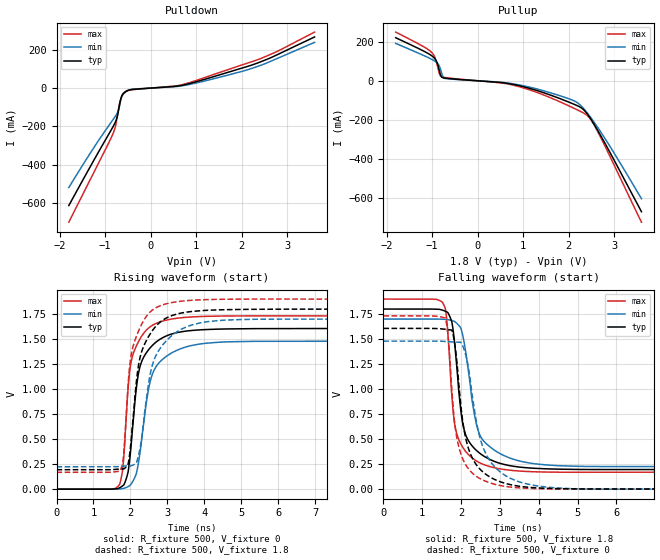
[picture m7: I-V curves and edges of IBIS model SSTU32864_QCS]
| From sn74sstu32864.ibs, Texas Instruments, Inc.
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[Model]   SSTU32864_QCS
Model_type  Output
Vref =   1.8
Rref =   1000
Cref =   30p
Vmeas =   0.9
| variable   typ   min   max
C_comp   4.54pF   3.63pF   5.50pF
| C_pullup   4.56pF   3.63pF   5.50pF
| C_pulldown   4.53pF   3.73pF   5.14pF
[Temperature Range]   40   85   0
| Ambient temperature   25   70   0
[Voltage range]   1.8   1.7   1.9
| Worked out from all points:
|   slope of the pulldown table from 0 to 0.27 V, typ, clamps not added: 60.6 ohm
|   slope of the pullup table from 0 to 0.27 V, typ, clamps not added: 59.5 ohm
|   rising waveform, R_fixture 500, V_fixture 0: 20-80 % time 327ps typ, 401ps min, 283ps max; typ from 0 V to 1.61 V
|   falling waveform, R_fixture 500, V_fixture 1.8: 20-80 % time 318ps typ, 405ps min, 261ps max; typ from 1.8 V to 0.195 V
|   rising waveform, R_fixture 500, V_fixture 1.8: 20-80 % time 396ps typ, 494ps min, 339ps max; typ from 0.195 V to 1.8 V
|   falling waveform, R_fixture 500, V_fixture 0: 20-80 % time 386ps typ, 519ps min, 301ps max; typ from 1.61 V to 0 V
[Pulldown]
| SSTU32864_QCS
|   Voltage   I(typ)   I(min)   I(max)
-1.8V     -613.5mA   -519.3mA   -700.4mA
-840mV    -206.5mA   -168.5mA   -244.1mA
-785mV    -181.7mA   -149.7mA   -207.8mA
-745mV    -156.6mA   -134.7mA   -162.6mA
-705mV    -112.3mA   -111.9mA   -105.3mA
-665mV    -63.66mA   -69.05mA   -61.98mA
-620mV    -34.48mA   -33.38mA   -36.65mA
-560mV    -20.07mA   -18.55mA   -21.69mA
-395mV    -6.837mA   -5.787mA   -8.284mA
880mV     25.3mA     20.45mA    30.74mA
2.26V     123.5mA    106mA      141mA
3.6V      267mA      238.9mA    292.5mA
[Pullup]
| SSTU32864_QCS
|   Voltage   I(typ)   I(min)   I(max)
-1.8V     219.6mA    190.8mA    248.4mA
-1.015V   128.7mA    110.2mA    145.7mA
-905mV    99.65mA    93.87mA    96.4mA
-840mV    50.49mA    74.02mA    36.2mA
-790mV    19.46mA    38.8mA     19.92mA
-700mV    13.37mA    11.24mA    16.34mA
870mV     -22.69mA   -19.2mA    -27.2mA
2.075V    -115.6mA   -97.82mA   -135.5mA
2.39V     -163.4mA   -158.5mA   -173.5mA
2.505V    -201.9mA   -193.6mA   -204.2mA
2.67V     -265.7mA   -248.8mA   -273.3mA
3.6V      -667.9mA   -601.5mA   -721.3mA
[Ramp]
| SSTU32864_QCS
| variable   typ   min   max
dV/dt_r   0.96/3.39E-10   0.89/4.20E-10   1.04/2.91E-10
dV/dt_f   0.96/3.29E-10   0.89/4.22E-10   1.04/2.68E-10
R_load = 500
[Rising Waveform]
| SSTU32864_QCS
R_fixture =   500
C_fixture =   0
L_fixture =   0
V_fixture =   0
V_fixture_min = 0
V_fixture_max = 0
|   Time   V(typ)   V(min)   V(max)
0s        395.3nV    2.664uV    74.81nV
1.705ns   13.27mV    2.411mV    45.03mV
1.805ns   37.73mV    6.765mV    252.2mV
1.935ns   166.3mV    25.1mV     994.5mV
2.09ns    736.1mV    95.15mV    1.368V
2.26ns    1.224V     364.5mV    1.502V
2.445ns   1.37V      897.7mV    1.595V
2.585ns   1.433V     1.139V     1.635V
3.285ns   1.567V     1.393V     1.71V
40ns      1.606V     1.479V     1.732V
[Falling Waveform]
| SSTU32864_QCS
R_fixture =   500
C_fixture =   0
L_fixture =   0
V_fixture =   1.8
V_fixture_min = 1.7
V_fixture_max = 1.9
|   Time   V(typ)   V(min)   V(max)
0s        1.8V       1.7V       1.9V
1.515ns   1.79V      1.698V     1.87V
1.625ns   1.773V     1.695V     1.714V
1.765ns   1.665V     1.685V     917.7mV
1.94ns    981.6mV    1.637V     495.4mV
2.11ns    549.8mV    1.395V     379.6mV
2.31ns    419.1mV    820.9mV    302.5mV
2.465ns   362.1mV    556.2mV    264.6mV
3.25ns    233.4mV    310.1mV    188mV
40ns      194.5mV    224.2mV    168.3mV
[Rising Waveform]
| SSTU32864_QCS
R_fixture =   500
C_fixture =   0
L_fixture =   0
V_fixture =   1.8
V_fixture_min = 1.7
V_fixture_max = 1.9
|   Time   V(typ)   V(min)   V(max)
0s        194.5mV    224.2mV    168.3mV
1.71ns    201.2mV    226.7mV    180.7mV
1.81ns    202.7mV    230.8mV    317.1mV
1.94ns    253mV      231.3mV    1.05V
2.015ns   467.1mV    233mV      1.329V
2.145ns   1.012V     256.9mV    1.51V
2.3ns     1.369V     497.8mV    1.645V
2.625ns   1.6V       1.276V     1.798V
3.38ns    1.761V     1.599V     1.879V
40ns      1.8V       1.7V       1.9V
[Falling Waveform]
| SSTU32864_QCS
R_fixture =   500
C_fixture =   0
L_fixture =   0
V_fixture =   0
V_fixture_min = 0
V_fixture_max = 0
|   Time   V(typ)   V(min)   V(max)
0s        1.606V     1.479V     1.732V
1.595ns   1.597V     1.476V     1.71V
1.68ns    1.593V     1.473V     1.467V
1.8ns     1.533V     1.471V     799.5mV
1.995ns   833.1mV    1.467V     349.4mV
2.195ns   398.8mV    1.198V     199.1mV
2.555ns   172.7mV    427.8mV    90.31mV
3.265ns   43.69mV    107.3mV    19.2mV
5.675ns   -411.7uV   -2.024mV   -1.034mV
40ns      395.2nV    2.665uV    74.78nV
